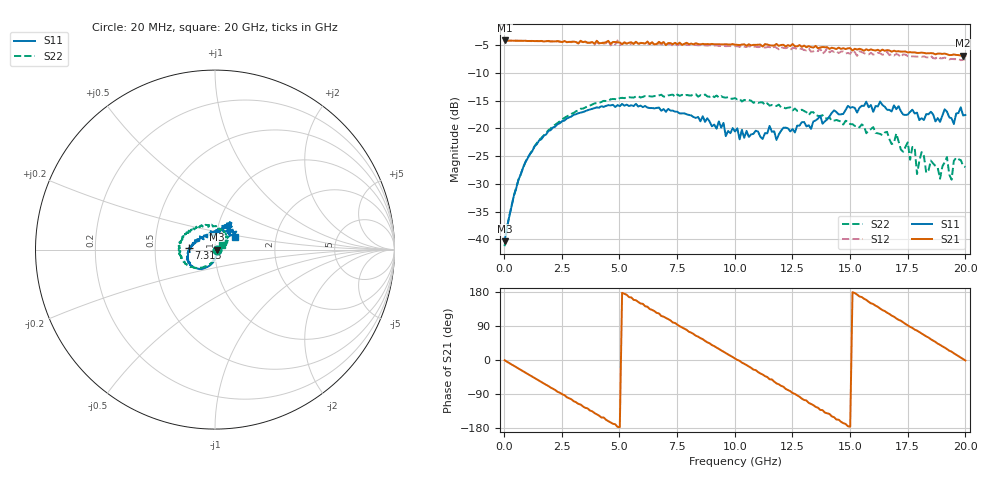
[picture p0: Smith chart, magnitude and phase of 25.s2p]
!Agilent Technologies,N5230A,US43500223,A.07.50.48
!Agilent N5230A: A.07.50.48
!Date: Wednesday, October 07, 2015 12:09:47
!Correction: S11(Full 2 Port(1,2))
!S21(Full 2 Port(1,2))
!S12(Full 2 Port(1,2))
!S22(Full 2 Port(1,2))
!S2P File: Measurements: S11, S21, S12, S22:
# Hz S  RI  R 50
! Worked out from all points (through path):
!   201 points, 20 MHz to 20 GHz, reference 50 ohm
!   highest |S21| = -4.10 dB at 20 MHz (marker M1); lowest = -6.8 dB at 19.9 GHz (marker M2)
!   group delay of S21, straight-line fit = 99.8 ps
!   lowest |S11| = -40.4 dB at 20 MHz (marker M3), VSWR 1.02, Z = 51 - j0.0747 ohm
!   |S11| at or under -10 dB: start of sweep to end of sweep
!   |S22| runs from -41.3 to -13.8 dB; largest |S21 - S12| = 0.094
!   S11 on the Smith chart (normalised r, x): 20 MHz: 1.02, -0.00; 7.313 GHz: 0.75, +0.01; 20 GHz: 1.24, +0.18
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2e7  0.00955 -0.000733  0.6233 -0.0079  0.6229 -0.00947  0.0086 -0.000898
1.019e9  -0.00215 -0.0537  0.494 -0.3698  0.4903 -0.3733  -0.00288 -0.0544
2.3177e9  -0.0471 -0.0985  0.0654 -0.6124  0.0528 -0.6119  -0.0595 -0.095
3.4166e9  -0.0923 -0.106  -0.3239 -0.507  -0.3486 -0.4879  -0.1121 -0.1012
4.9151e9  -0.1425 -0.0778  -0.598 -0.0358  -0.623 -0.0189  -0.1689 -0.0674
6.7133e9  -0.1532 -0.0188  -0.3287 0.5091  -0.2906 0.5093  -0.1982 -0.0161
7.3127e9  -0.1448 0.00704  -0.0899 0.5698  -0.0555 0.5565  -0.202 -0.00237
8.6114e9  -0.1237 0.0365  0.3334 0.4763  0.3596 0.4394  -0.1944 0.0374
1.001e10  -0.0582 0.0735  0.5693 0.0374  0.5547 -0.00414  -0.1683 0.0838
1.18082e10  -0.00394 0.0788  0.2747 -0.5118  0.2104 -0.4936  -0.1034 0.1217
1.34066e10  0.0246 0.1132  -0.2621 -0.4694  -0.275 -0.4148  -0.0196 0.1388
1.51049e10  0.0776 0.1356  -0.5058 0.00947  -0.5047 0.0528  0.0502 0.0973
1.67033e10  0.0722 0.1284  -0.2654 0.4314  -0.1993 0.414  0.0675 0.0431
1.78022e10  0.0812 0.1096  0.0819 0.48  0.1111 0.4331  0.0621 0.0256
1.79021e10  0.0791 0.1143  0.1038 0.4701  0.1358 0.4237  0.0342 0.0181
1.81019e10  0.0697 0.1024  0.1654 0.4552  0.1856 0.4029  0.0482 0.0377
1.89011e10  0.0684 0.0922  0.3641 0.3046  0.3613 0.2344  0.0307 0.0171
1.92008e10  0.1021 0.0987  0.41 0.2258  0.4003 0.1609  0.0488 0.0257
1.94006e10  0.0918 0.0827  0.427 0.1734  0.4096 0.1127  0.0293 0.0181
1.96004e10  0.0833 0.1078  0.4482 0.1105  0.4179 0.0632  0.0426 0.0338
1.99001e10  0.105 0.0786  0.455 0.0215  0.4171 -0.0176  0.0426 0.0175
2e10  0.1115 0.0712  0.4556 -0.00928  0.4176 -0.0579  0.0376 0.0244
